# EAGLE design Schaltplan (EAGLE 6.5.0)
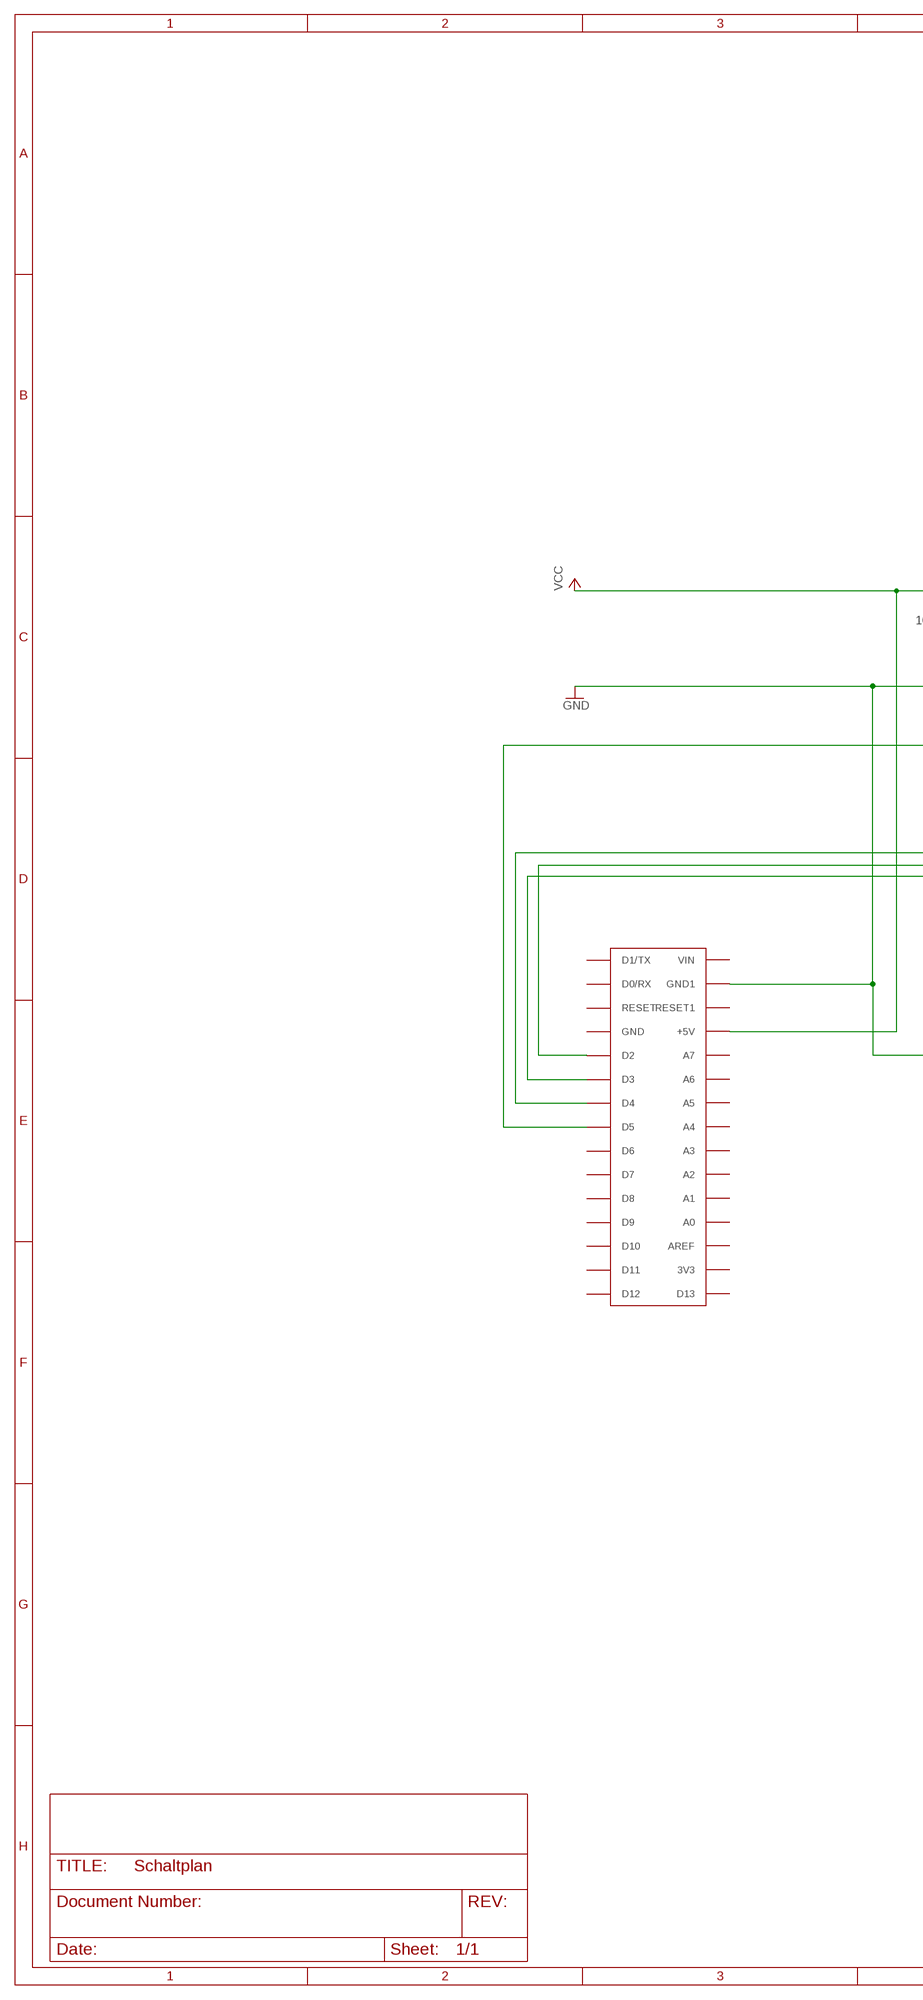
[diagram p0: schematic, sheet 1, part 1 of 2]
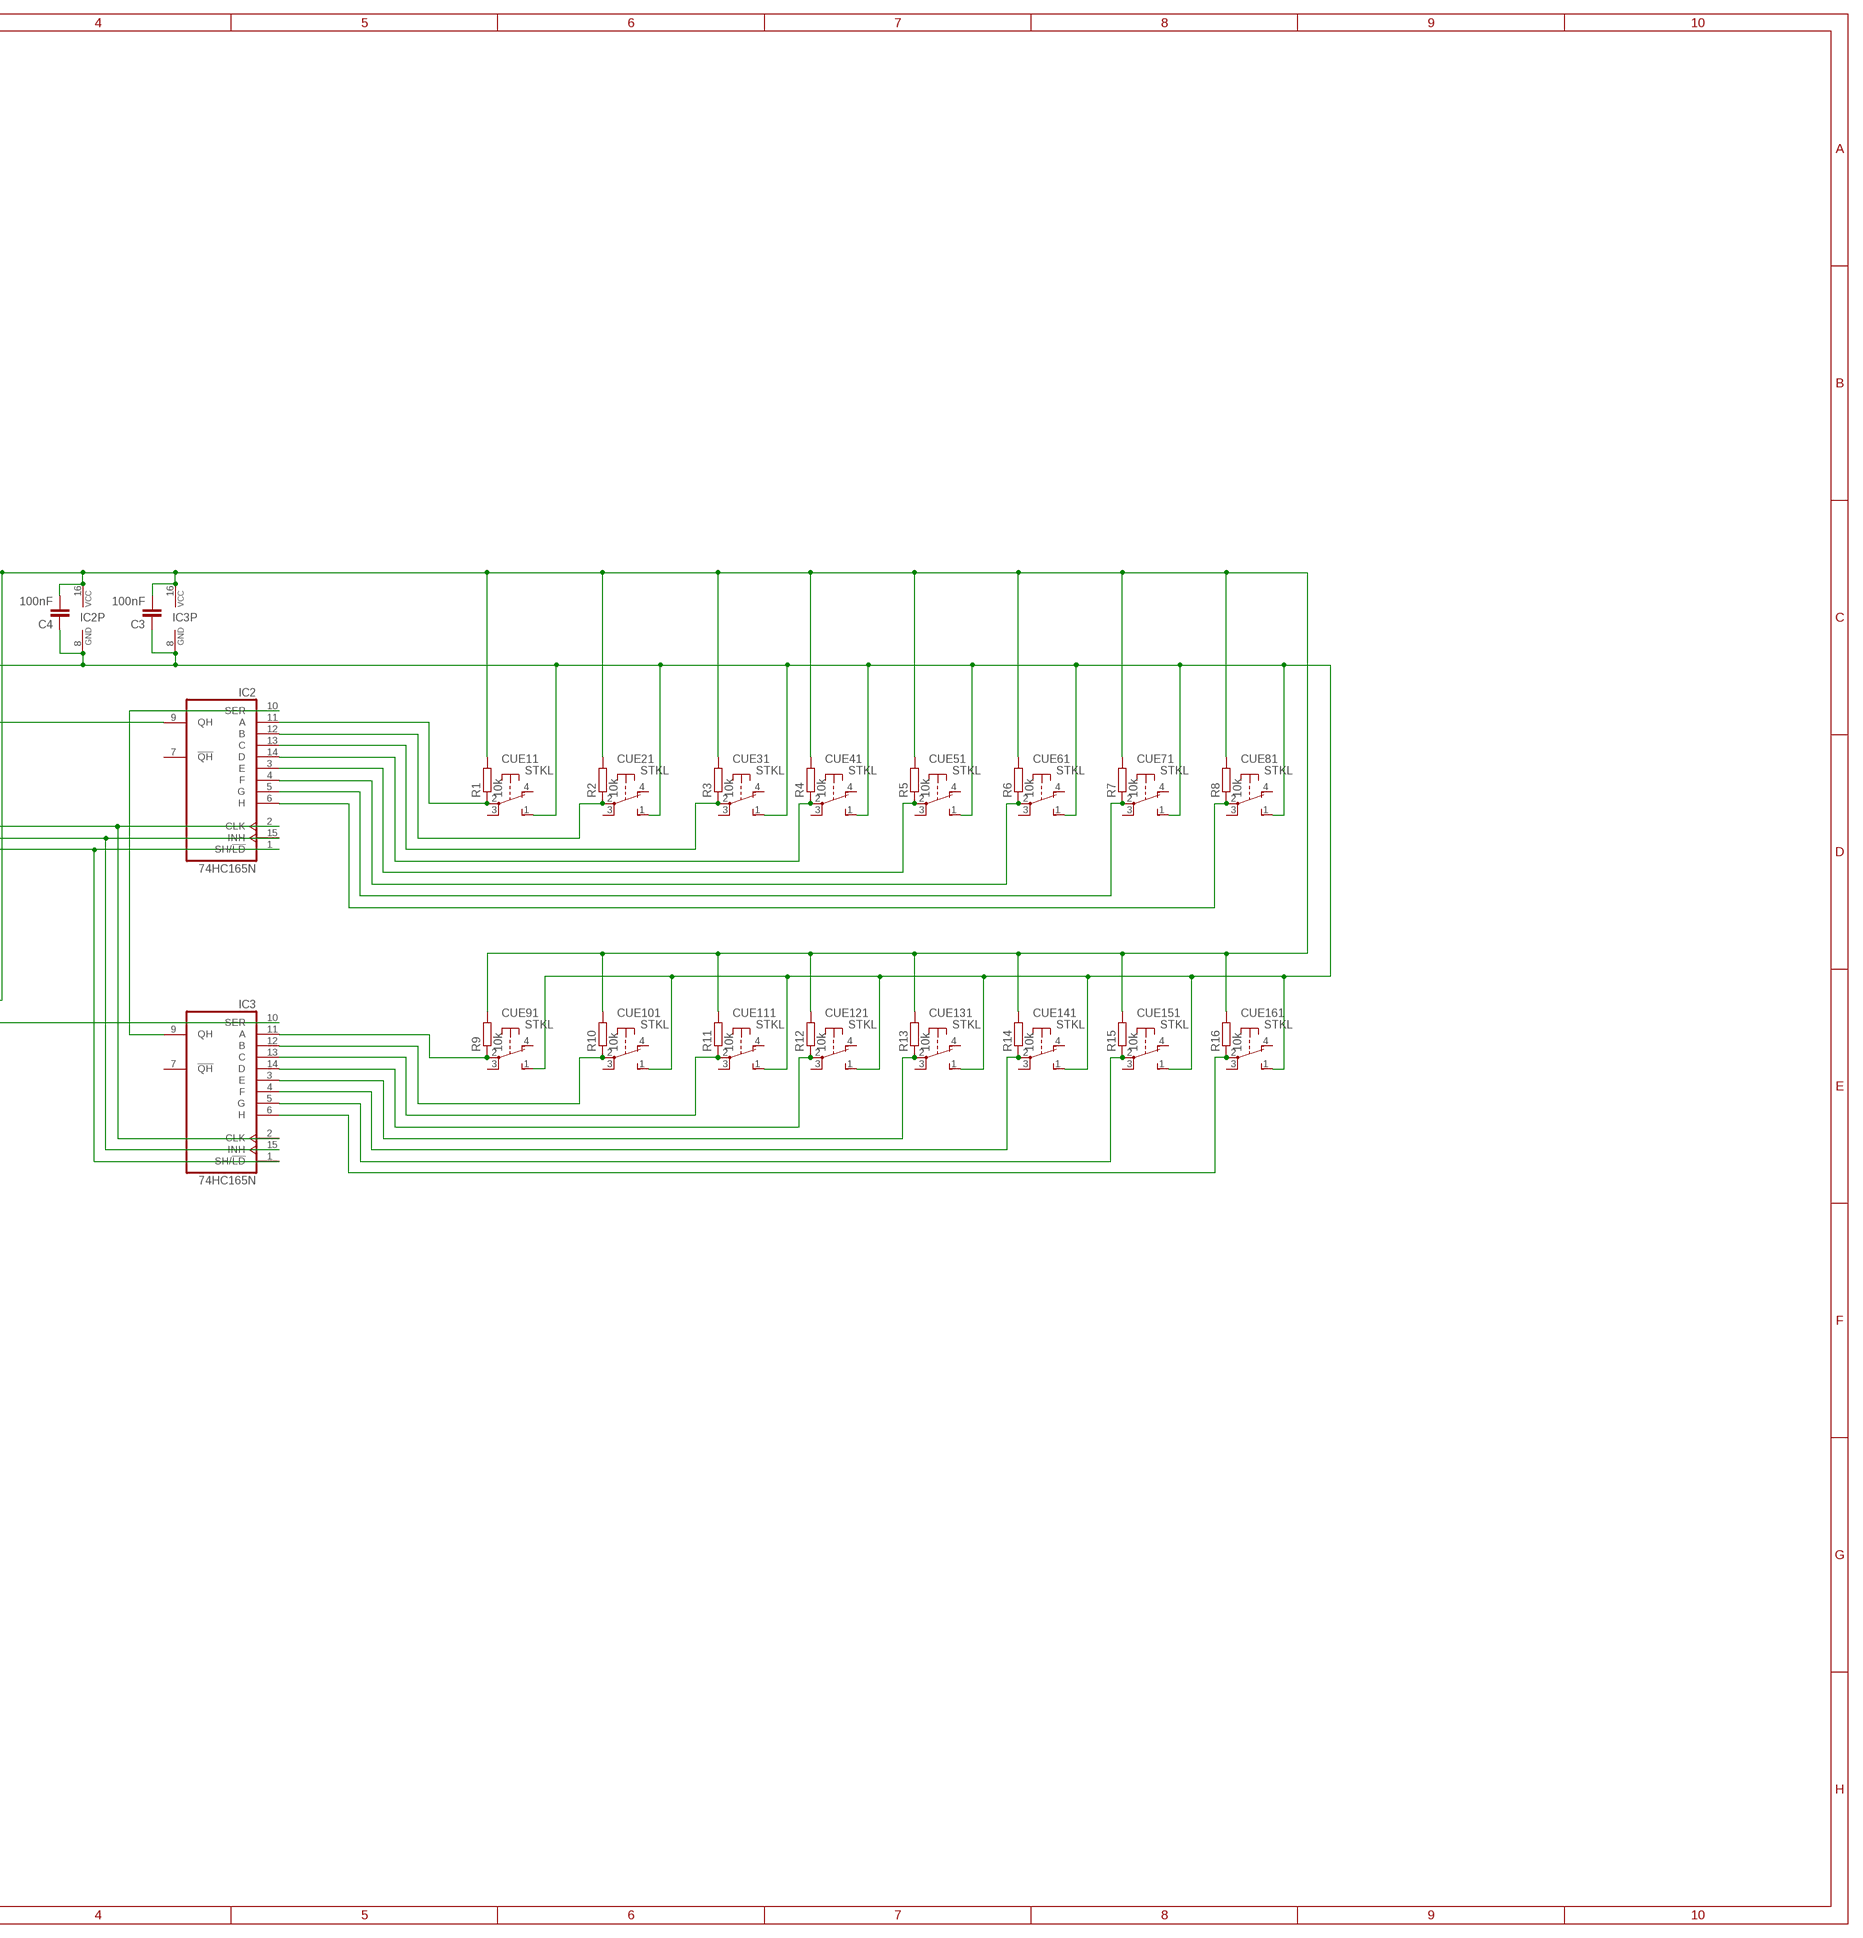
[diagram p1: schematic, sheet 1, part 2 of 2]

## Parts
C3  100nF  C-EUC1206  [C1206]
C4  100nF  C-EUC1206  [C1206]
CUE1  STKL  [STKL]
CUE2  STKL  [STKL]
CUE3  STKL  [STKL]
CUE4  STKL  [STKL]
CUE5  STKL  [STKL]
CUE6  STKL  [STKL]
CUE7  STKL  [STKL]
CUE8  STKL  [STKL]
CUE9  STKL  [STKL]
CUE10  STKL  [STKL]
CUE11  STKL  [STKL]
CUE12  STKL  [STKL]
CUE13  STKL  [STKL]
CUE14  STKL  [STKL]
CUE15  STKL  [STKL]
CUE16  STKL  [STKL]
IC2  74HC165N  [DIL16]
IC3  74HC165N  [DIL16]
R1  10k  R-EU_R1206  [R1206]
R2  10k  R-EU_R1206  [R1206]
R3  10k  R-EU_R1206  [R1206]
R4  10k  R-EU_R1206  [R1206]
R5  10k  R-EU_R1206  [R1206]
R6  10k  R-EU_R1206  [R1206]
R7  10k  R-EU_R1206  [R1206]
R8  10k  R-EU_R1206  [R1206]
R9  10k  R-EU_R1206  [R1206]
R10  10k  R-EU_R1206  [R1206]
R11  10k  R-EU_R1206  [R1206]
R12  10k  R-EU_R1206  [R1206]
R13  10k  R-EU_R1206  [R1206]
R14  10k  R-EU_R1206  [R1206]
R15  10k  R-EU_R1206  [R1206]
R16  10k  R-EU_R1206  [R1206]
U$1  ARDUINONANO1,1MM-BOHRUNG  [PDIP-32GROSSE-BOHRUNG]

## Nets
GND: C3.1 C4.1 CUE1.1(1:S) CUE2.1(1:S) CUE3.1(1:S) CUE4.1(1:S) CUE5.1(1:S) CUE6.1(1:S) CUE7.1(1:S) CUE8.1(1:S) CUE9.1(1:S) CUE10.1(1:S) CUE11.1(1:S) CUE12.1(1:S) CUE13.1(1:S) CUE14.1(1:S) CUE15.1(1:S) CUE16.1(1:S) IC2.8(GND) IC3.8(GND) IC3.10(SER) U$1.GND1
N$1: CUE1.2(1:P) IC2.11(A) R1.1
N$2: CUE2.2(1:P) IC2.12(B) R2.1
N$3: CUE3.2(1:P) IC2.13(C) R3.1
N$4: CUE4.2(1:P) IC2.14(D) R4.1
N$5: IC2.15(INH) IC3.15(INH) U$1.D2
N$6: IC2.2(CLK) IC3.2(CLK) U$1.D4
N$7: CUE12.2(1:P) IC3.14(D) R12.1
N$8: IC2.9(QH) U$1.D5
N$9: IC2.10(SER) IC3.9(QH)
N$15: CUE5.2(1:P) IC2.3(E) R5.1
N$16: CUE6.2(1:P) IC2.4(F) R6.1
N$17: CUE7.2(1:P) IC2.5(G) R7.1
N$18: CUE8.2(1:P) IC2.6(H) R8.1
N$23: CUE9.2(1:P) IC3.11(A) R9.1
N$24: CUE10.2(1:P) IC3.12(B) R10.1
N$25: CUE11.2(1:P) IC3.13(C) R11.1
N$27: CUE13.2(1:P) IC3.3(E) R13.1
N$28: CUE14.2(1:P) IC3.4(F) R14.1
N$29: CUE15.2(1:P) IC3.5(G) R15.1
N$30: CUE16.2(1:P) IC3.6(H) R16.1
N$70: IC2.1(SH/!LD) IC3.1(SH/!LD) U$1.D3
VCC: C3.2 C4.2 IC2.16(VCC) IC3.16(VCC) R1.2 R2.2 R3.2 R4.2 R5.2 R6.2 R7.2 R8.2 R9.2 R10.2 R11.2 R12.2 R13.2 R14.2 R15.2 R16.2 U$1.+5V
Unconnected: CUE1.3(1:P) CUE1.4(1:O) CUE1.+(D1:A) CUE1.-(D1:C) CUE2.3(1:P) CUE2.4(1:O) CUE2.+(D1:A) CUE2.-(D1:C) CUE3.3(1:P) CUE3.4(1:O) CUE3.+(D1:A) CUE3.-(D1:C) CUE4.3(1:P) CUE4.4(1:O) CUE4.+(D1:A) CUE4.-(D1:C) CUE5.3(1:P) CUE5.4(1:O) CUE5.+(D1:A) CUE5.-(D1:C) CUE6.3(1:P) CUE6.4(1:O) CUE6.+(D1:A) CUE6.-(D1:C) CUE7.3(1:P) CUE7.4(1:O) CUE7.+(D1:A) CUE7.-(D1:C) CUE8.3(1:P) CUE8.4(1:O) CUE8.+(D1:A) CUE8.-(D1:C) CUE9.3(1:P) CUE9.4(1:O) CUE9.+(D1:A) CUE9.-(D1:C) CUE10.3(1:P) CUE10.4(1:O) CUE10.+(D1:A) CUE10.-(D1:C) CUE11.3(1:P) CUE11.4(1:O) CUE11.+(D1:A) CUE11.-(D1:C) CUE12.3(1:P) CUE12.4(1:O) CUE12.+(D1:A) CUE12.-(D1:C) CUE13.3(1:P) CUE13.4(1:O) CUE13.+(D1:A) CUE13.-(D1:C) CUE14.3(1:P) CUE14.4(1:O) CUE14.+(D1:A) CUE14.-(D1:C) CUE15.3(1:P) CUE15.4(1:O) CUE15.+(D1:A) CUE15.-(D1:C) CUE16.3(1:P) CUE16.4(1:O) CUE16.+(D1:A) CUE16.-(D1:C) IC2.7(!QH) IC3.7(!QH) U$1.3V3 U$1.A0 U$1.A1 U$1.A2 U$1.A3 U$1.A4 U$1.A5 U$1.A6 U$1.A7 U$1.AREF U$1.D0/RX U$1.D1/TX U$1.D6 U$1.D7 U$1.D8 U$1.D9 U$1.D10 U$1.D11 U$1.D12 U$1.D13 U$1.GND U$1.RESET U$1.RESET1 U$1.VIN

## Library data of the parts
C3 C4 = rcl:C-EU: CAPACITOR, European symbol
CUE1-CUE16 = switch-misc:STKL: SWITCH
IC2 IC3 = 74xx-eu:74*165: 8-bit parallel load SHIFT REGISTER
R1-R16 = rcl:R-EU_: RESISTOR, European symbol
U$1 = arduino:ARDUINONANO

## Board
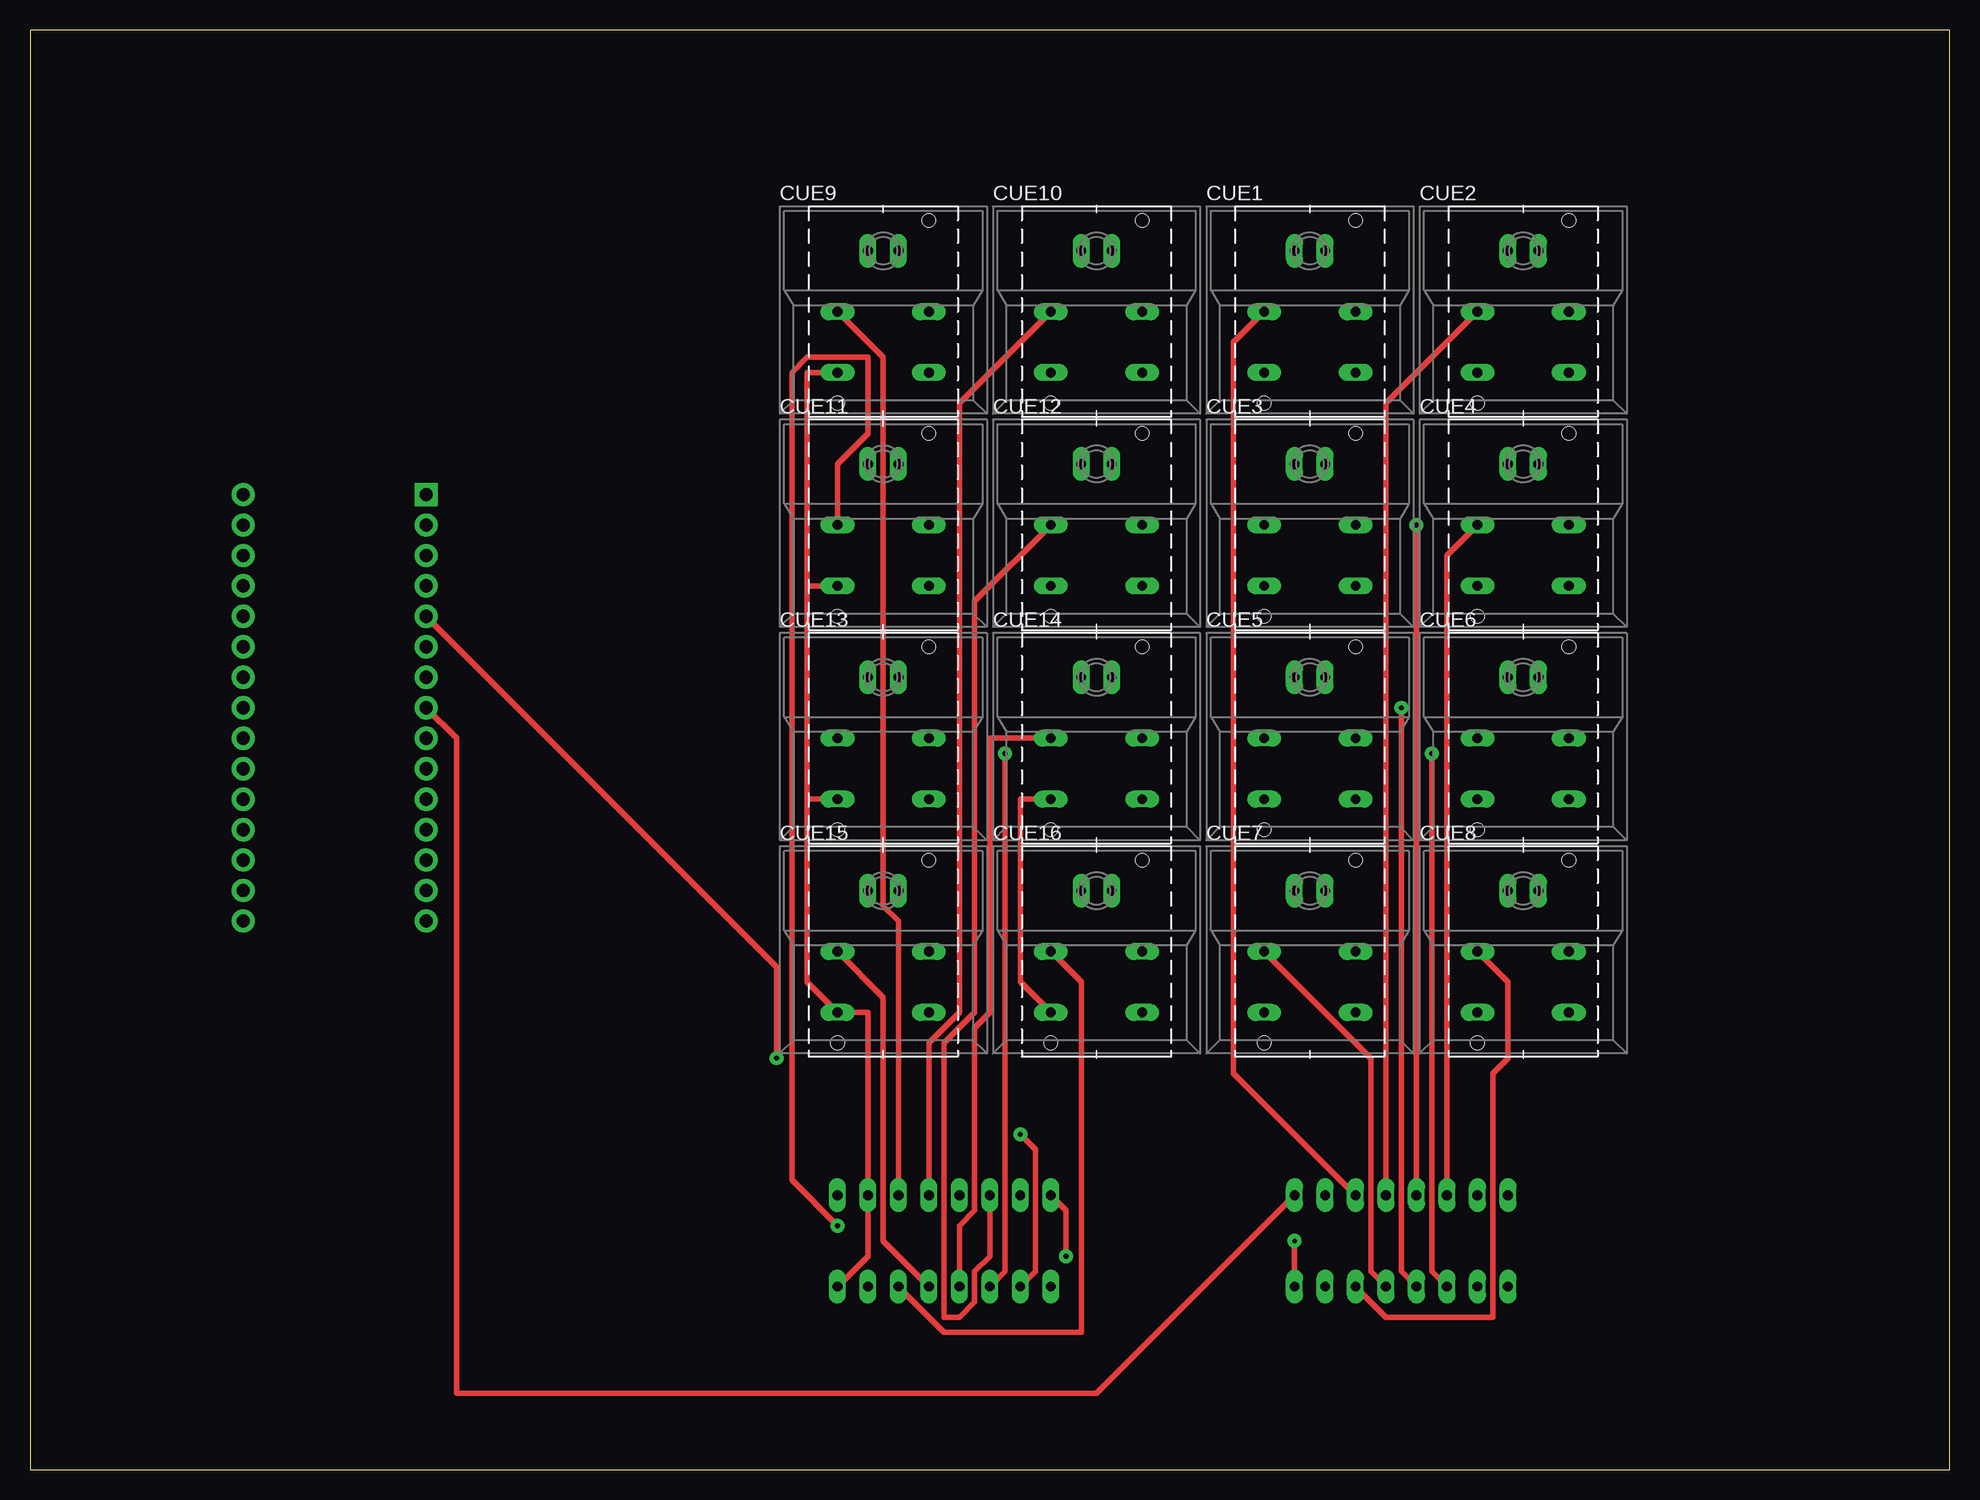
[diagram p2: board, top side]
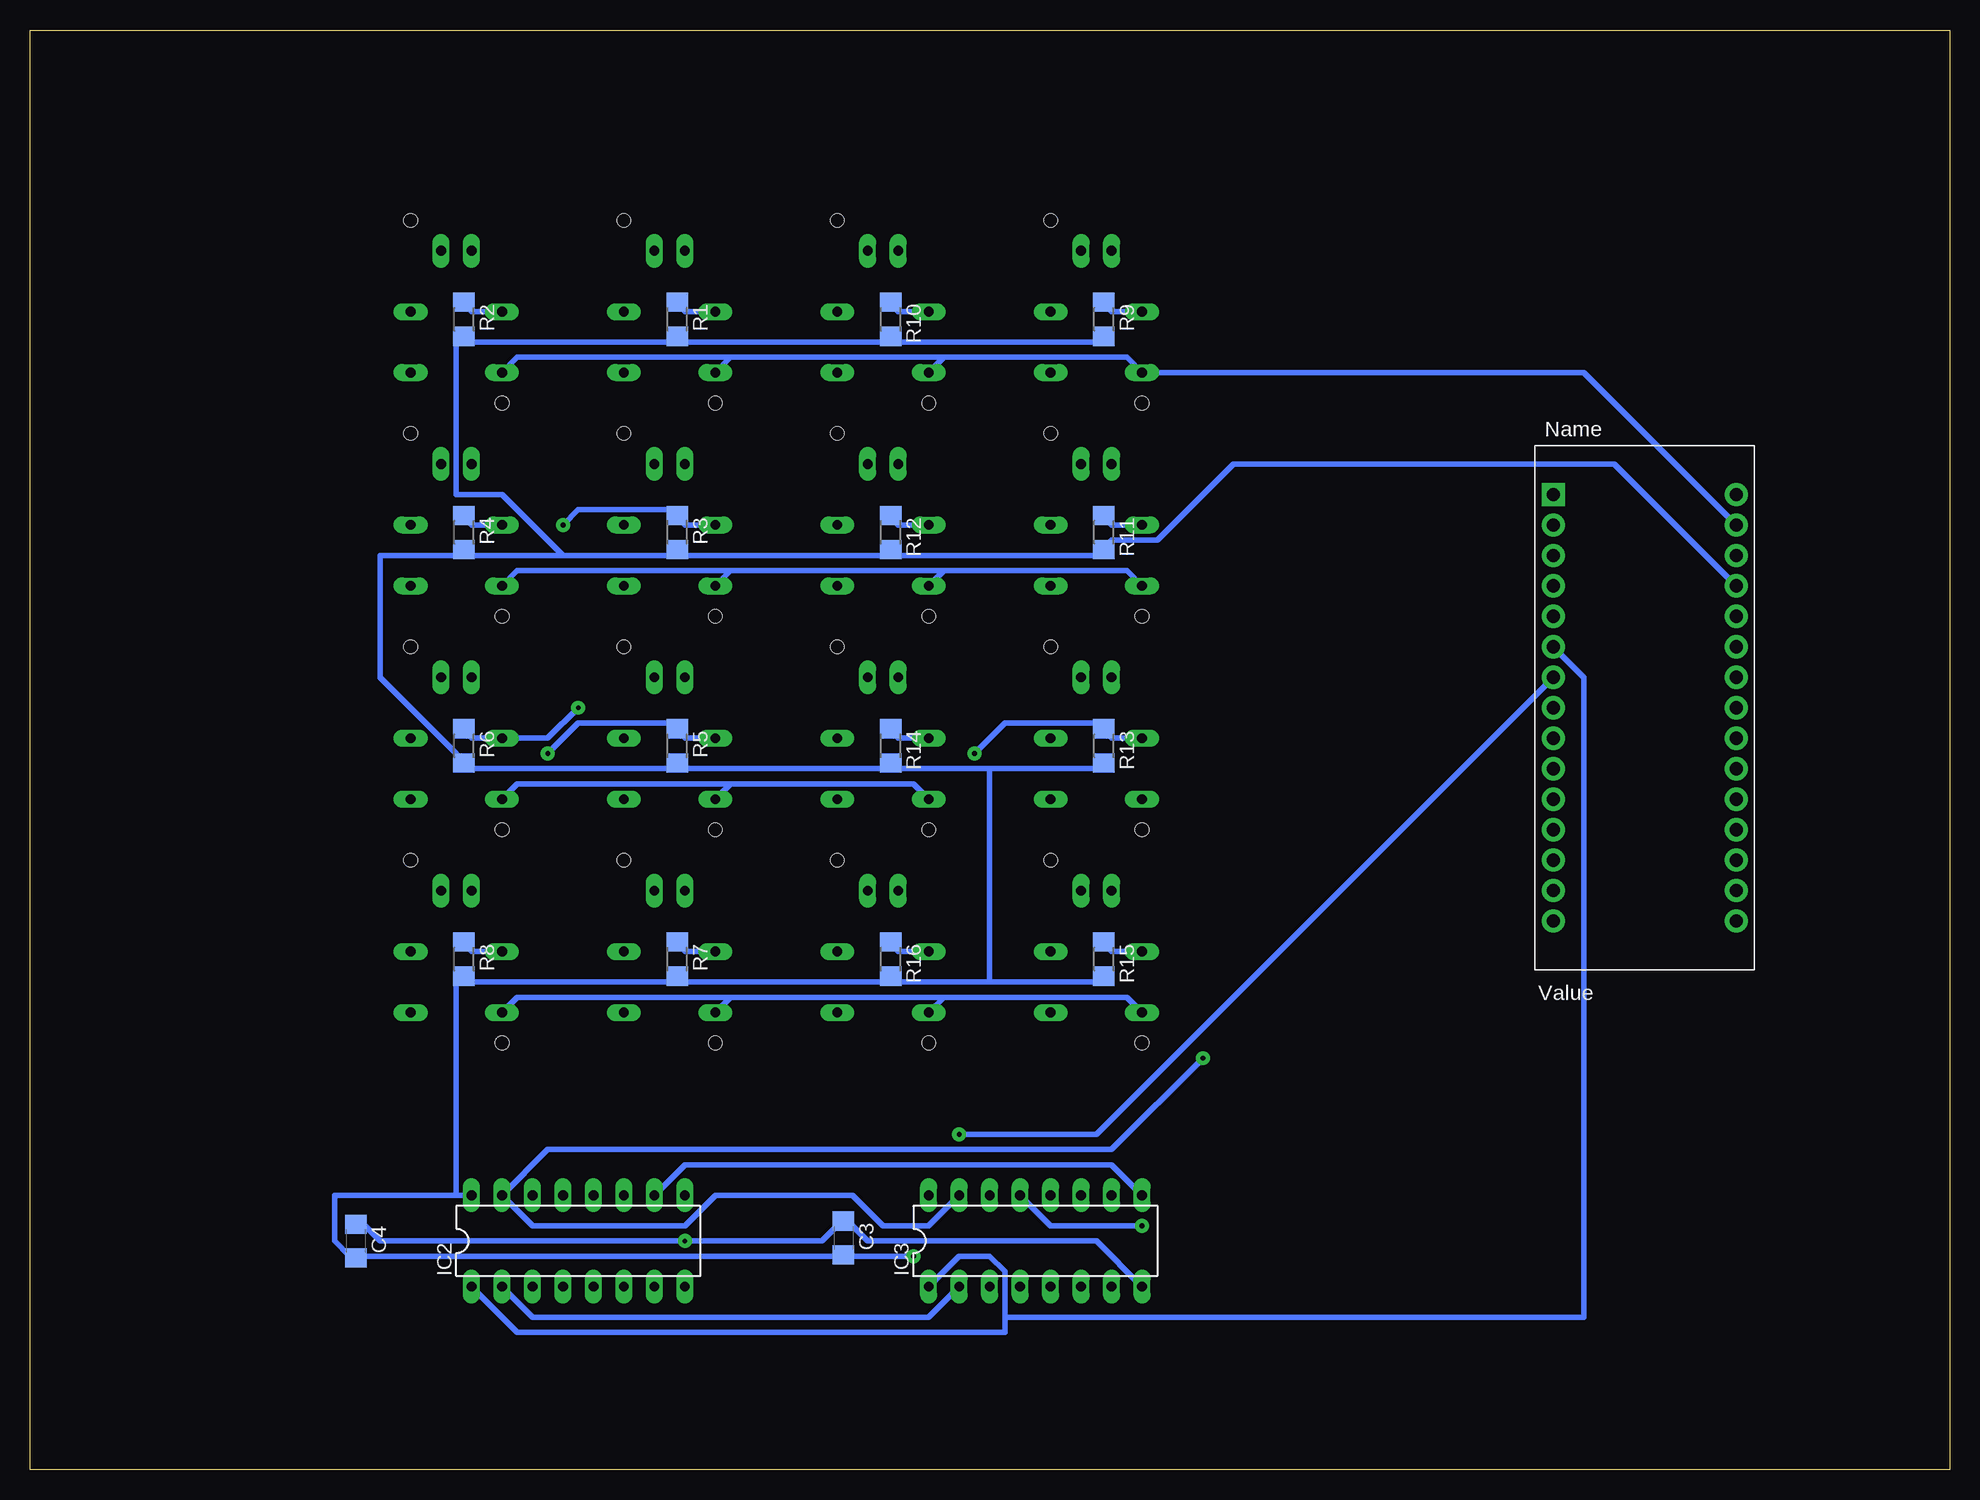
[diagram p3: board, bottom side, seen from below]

Size 160 x 120 mm. Coordinates in mm from the lower left corner, seen from the top.
Outline: 0,0 160,0 160,120 0,120 0,0
Copper layers (1*16): Top 0.035mm / dielectric 1.5mm / Bottom 0.035mm
Design rules "HTWG Sinnvoll": minimum track width 18mil, minimum drill 0.4mm, track to track 12mil, track to pad 12mil, pad to pad 18mil, via to via 18mil, smd to smd 18mil, copper to edge 40mil, drill to drill 8mil, minimum pad ring 12mil, minimum via ring 15mil, stop-mask expansion 4mil, vias tented up to drill 0mil, thermal gap 10mil

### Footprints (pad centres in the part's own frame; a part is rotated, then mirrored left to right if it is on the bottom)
C1206 = smd 1.6 x 1.8: 1 -1.4,0; 2 1.4,0
STKL = drill 0.813 long: 1 -3.81,-5.08; 2 -3.81,0; 3 3.81,0; 4 3.81,-5.08; + -1.27,5.08; - 1.27,5.08 | hole 1.118: 3.81,7.62; -3.81,-7.62
DIL16 = drill 0.813 long: 1 -8.89,-3.81; 2 -6.35,-3.81; 3 -3.81,-3.81; 4 -1.27,-3.81; 5 1.27,-3.81; 6 3.81,-3.81; 7 6.35,-3.81; 8 8.89,-3.81; 9 8.89,3.81; 10 6.35,3.81; 11 3.81,3.81; 12 1.27,3.81; 13 -1.27,3.81; 14 -3.81,3.81; 15 -6.35,3.81; 16 -8.89,3.81
R1206 = smd 1.6 x 1.803: 1 -1.422,0; 2 1.422,0
PDIP-32GROSSE-BOHRUNG = drill 1.1 pad 1.93: 3V3 15.24,-35.56; +5V 15.24,-10.16; A0 15.24,-30.48; A1 15.24,-27.94; A2 15.24,-25.4; A3 15.24,-22.86; A4 15.24,-20.32; A5 15.24,-17.78; A6 15.24,-15.24; A7 15.24,-12.7; AREF 15.24,-33.02; D0/RX 0,-5.08; D2 0,-12.7; D3 0,-15.24; D4 0,-17.78; D5 0,-20.32; D6 0,-22.86; D7 0,-25.4; D8 0,-27.94; D9 0,-30.48; D10 0,-33.02; D11 0,-35.56; D12 0,-38.1; D13 15.24,-38.1; GND 0,-10.16; GND1 15.24,-5.08; RESET 0,-7.62; RESET1 15.24,-7.62; VIN 15.24,-2.54 | drill 1.1 pad 1.93 square: D1/TX 0,-2.54

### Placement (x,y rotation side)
C3  92.2,19.3 270 bottom
C4  132.84,19.05 270 bottom
CUE1  106.68,96.52 0 top
CUE2  124.46,96.52 0 top
CUE3  106.68,78.74 0 top
CUE4  124.46,78.74 0 top
CUE5  106.68,60.96 0 top
CUE6  124.46,60.96 0 top
CUE7  106.68,43.18 0 top
CUE8  124.46,43.18 0 top
CUE9  71.12,96.52 0 top
CUE10  88.9,96.52 0 top
CUE11  71.12,78.74 0 top
CUE12  88.9,78.74 0 top
CUE13  71.12,60.96 0 top
CUE14  88.9,60.96 0 top
CUE15  71.12,43.18 0 top
CUE16  88.9,43.18 0 top
IC2  114.3,19.05 0 bottom
IC3  76.2,19.05 0 bottom
R1  106.05,95.89 270 bottom
R2  123.83,95.89 270 bottom
R3  106.05,78.11 270 bottom
R4  123.83,78.11 270 bottom
R5  106.05,60.33 270 bottom
R6  123.83,60.33 270 bottom
R7  106.05,42.55 270 bottom
R8  123.83,42.55 270 bottom
R9  70.48,95.89 270 bottom
R10  88.27,95.89 270 bottom
R11  70.48,78.11 270 bottom
R12  88.27,78.11 270 bottom
R13  70.48,60.33 270 bottom
R14  88.27,60.33 270 bottom
R15  70.48,42.55 270 bottom
R16  88.27,42.55 270 bottom
U$1  33.02,83.82 0 bottom

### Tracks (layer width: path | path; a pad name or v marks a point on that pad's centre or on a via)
GND  (via drill 0.4)
  Top 0.457: v105.41,19.05 IC2.8 | 64.77,55.88 CUE13.1 | 64.77,55.88 64.77,40.64 CUE15.1 69.85,38.1 IC3.10 69.85,17.78 IC3.8 | 64.77,73.66 CUE11.1 | 64.77,55.88 64.77,73.66 | CUE9.1 64.77,91.44 64.77,73.66 | CUE14.1 82.55,55.88 82.55,40.64 CUE16.1
  Bottom 0.457: IC3.8 71.12,19.05 90.17,19.05 91.44,20.32 C3.1 92.71,20.32 93.98,19.05 v105.41,19.05 130.81,19.05 132.08,20.32 C4.1 | CUE14.1 86.36,57.15 101.6,57.15 | CUE5.1 101.6,57.15 | CUE6.1 119.38,57.15 101.6,57.15 | 83.82,39.37 CUE16.1 | 83.82,39.37 68.58,39.37 CUE15.1 | 101.6,39.37 CUE7.1 | 83.82,39.37 101.6,39.37 | CUE8.1 119.38,39.37 101.6,39.37 | 83.82,74.93 CUE12.1 | 83.82,74.93 68.58,74.93 CUE11.1 | 101.6,74.93 CUE3.1 | 83.82,74.93 101.6,74.93 | CUE4.1 119.38,74.93 101.6,74.93 | 83.82,92.71 CUE10.1 | 83.82,92.71 68.58,92.71 CUE9.1 30.48,91.44 U$1.GND1 | 101.6,92.71 CUE1.1 | 83.82,92.71 101.6,92.71 | CUE2.1 119.38,92.71 101.6,92.71
N$1
  Top 0.457: IC2.11 100.33,33.02 100.33,93.98 CUE1.2
  Bottom 0.457: CUE1.2 105.41,96.52 R1.1
N$2
  Top 0.457: IC2.12 113.03,88.9 CUE2.2
  Bottom 0.457: CUE2.2 123.19,96.52 R2.1
N$3  (via drill 0.4)
  Top 0.457: v115.57,78.74 IC2.13
  Bottom 0.457: CUE3.2 105.41,78.74 R3.1 106.68,80.01 114.3,80.01 v115.57,78.74
N$4
  Top 0.457: IC2.14 118.11,76.2 CUE4.2
  Bottom 0.457: CUE4.2 123.19,78.74 R4.1
N$5  (via drill 0.4)
  Top 0.457: U$1.D2 62.23,41.91 v62.23,34.29
  Bottom 0.457: IC3.15 85.09,20.32 88.9,20.32 91.44,22.86 102.87,22.86 105.41,20.32 118.11,20.32 IC2.15 116.84,26.67 69.85,26.67 v62.23,34.29
N$6  (via drill 0.4)
  Top 0.457: v82.55,27.94 83.82,26.67 83.82,16.51 IC3.2
  Bottom 0.457: IC3.2 85.09,12.7 118.11,12.7 IC2.2 | U$1.D4 71.12,27.94 v82.55,27.94
N$7
  Top 0.457: IC3.14 80.01,17.78 78.74,16.51 78.74,13.97 77.47,12.7 76.2,12.7 76.2,35.56 78.74,38.1 78.74,72.39 CUE12.2
  Bottom 0.457: CUE12.2 87.63,78.74 R12.1
N$8
  Top 0.457: IC2.9 88.9,6.35 35.56,6.35 35.56,60.96 U$1.D5
N$9
  Bottom 0.457: IC3.9 69.85,25.4 105.41,25.4 IC2.10
N$15  (via drill 0.4)
  Top 0.457: IC2.3 116.84,16.51 v116.84,59.69
  Bottom 0.457: CUE5.2 105.41,60.96 R5.1 106.68,62.23 114.3,62.23 v116.84,59.69
N$16  (via drill 0.4)
  Top 0.457: IC2.4 114.3,16.51 v114.3,63.5
  Bottom 0.457: R6.1 123.19,60.96 CUE6.2 116.84,60.96 v114.3,63.5
N$17
  Top 0.457: IC2.5 111.76,16.51 111.76,34.29 CUE7.2
  Bottom 0.457: CUE7.2 105.41,43.18 R7.1
N$18
  Top 0.457: IC2.6 113.03,12.7 121.92,12.7 121.92,33.02 123.19,34.29 123.19,40.64 CUE8.2
  Bottom 0.457: CUE8.2 123.19,43.18 R8.1
N$23
  Top 0.457: IC3.11 72.39,45.72 71.12,46.99 71.12,92.71 CUE9.2
  Bottom 0.457: CUE9.2 69.85,96.52 R9.1
N$24
  Top 0.457: IC3.12 74.93,35.56 77.47,38.1 77.47,88.9 CUE10.2
  Bottom 0.457: CUE10.2 87.63,96.52 R10.1
N$25  (via drill 0.4)
  Top 0.457: v67.31,20.32 63.5,24.13 63.5,91.44 64.77,92.71 69.85,92.71 69.85,86.36 67.31,83.82 CUE11.2
  Bottom 0.457: CUE11.2 69.85,78.74 R11.1 | IC3.13 74.93,20.32 v67.31,20.32
N$27  (via drill 0.4)
  Top 0.457: IC3.3 81.28,16.51 v81.28,59.69
  Bottom 0.457: CUE13.2 69.85,60.96 R13.1 71.12,62.23 78.74,62.23 v81.28,59.69
N$28
  Top 0.457: IC3.4 77.47,20.32 78.74,21.59 78.74,36.83 80.01,38.1 80.01,60.96 CUE14.2
  Bottom 0.457: CUE14.2 87.63,60.96 R14.1
N$29
  Top 0.457: IC3.5 71.12,19.05 71.12,39.37 CUE15.2
  Bottom 0.457: CUE15.2 69.85,43.18 R15.1
N$30
  Top 0.457: IC3.6 76.2,11.43 87.63,11.43 87.63,40.64 CUE16.2
  Bottom 0.457: CUE16.2 87.63,43.18 R16.1
N$70
  Bottom 0.457: IC3.1 82.55,17.78 80.01,17.78 78.74,16.51 78.74,12.7 | 78.74,12.7 78.74,11.43 119.38,11.43 IC2.1 | U$1.D3 30.48,66.04 30.48,12.7 78.74,12.7
VCC  (via drill 0.4)
  Top 0.457: IC3.16 86.36,21.59 v86.36,17.78
  Bottom 0.457: 80.01,58.42 87.63,58.42 R14.2 88.9,58.42 105.41,58.42 R5.2 106.68,58.42 123.19,58.42 R6.2 124.46,59.69 130.81,66.04 130.81,76.2 124.46,76.2 R4.2 123.19,76.2 115.57,76.2 | 80.01,58.42 71.12,58.42 R13.2 | 80.01,40.64 87.63,40.64 R16.2 88.9,40.64 105.41,40.64 R7.2 106.68,40.64 123.19,40.64 R8.2 124.46,40.64 124.46,22.86 | 80.01,40.64 71.12,40.64 R15.2 | IC2.16 124.46,22.86 | 124.46,22.86 134.62,22.86 134.62,19.05 133.35,17.78 C4.2 132.08,17.78 92.71,17.78 C3.2 91.44,17.78 v86.36,17.78 | 80.01,40.64 80.01,58.42 | R9.2 71.12,93.98 87.63,93.98 R10.2 88.9,93.98 105.41,93.98 R1.2 106.68,93.98 123.19,93.98 R2.2 124.46,93.98 124.46,81.28 120.65,81.28 115.57,76.2 | 115.57,76.2 106.68,76.2 R3.2 105.41,76.2 88.9,76.2 R12.2 87.63,76.2 71.12,76.2 R11.2 69.85,77.47 66.04,77.47 59.69,83.82 27.94,83.82 U$1.+5V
